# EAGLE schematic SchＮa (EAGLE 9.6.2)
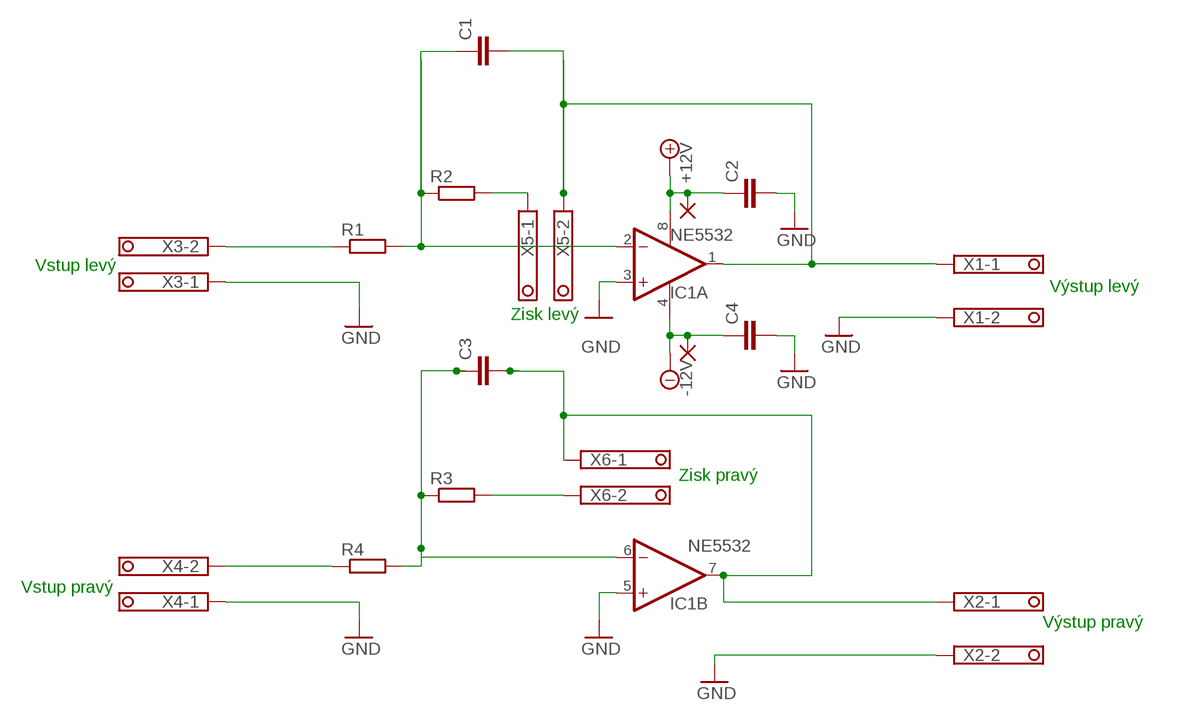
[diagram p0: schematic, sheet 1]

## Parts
+12V  1,6/0,8  [1,6/0,8]
-12V  1,6/0,8  [1,6/0,8]
C1  C-EUC1206  [C1206]
C2  C-EUC1206  [C1206]
C3  C-EUC1206  [C1206]
C4  C-EUC1206  [C1206]
IC1  NE5532  NE5532N  [DIL08]
R1  R-EU_M1206  [M1206]
R2  R-EU_M1206  [M1206]
R3  R-EU_M1206  [M1206]
R4  R-EU_M1206  [M1206]
X1  1751248  [1751248]
X2  1751248  [1751248]
X3  1751248  [1751248]
X4  1751248  [1751248]
X5  1751248  [1751248]
X6  1751248  [1751248]

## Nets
+12V: +12V.1(P) C2.1 IC1.8(P:V+)
-12V: -12V.1(P) C4.1 IC1.4(P:V-)
GND: C2.2 C4.2 IC1.3(A:+IN) IC1.5(B:+IN) X1.2 X2.2 X3.1 X4.1
N$1: C1.1 IC1.2(A:-IN) R1.2 R2.1
N$2: C3.1 IC1.6(B:-IN) R3.1 R4.2
N$3: R2.2 X5.1
N$4: R3.2 X6.2
N$5: C1.2 IC1.1(A:OUT) X1.1 X5.2
N$6: C3.2 IC1.7(B:OUT) X2.1 X6.1
N$7: R1.1 X3.2
N$8: R4.1 X4.2

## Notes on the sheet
- Vstup levý
- Výstup levý
- Zisk levý
- Zisk pravý
- Vstup pravý
- Výstup pravý

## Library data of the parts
+12V -12V = wirepad:1,6/0,8: THROUGH-HOLE PAD
C1-C4 = rcl:C-EU: CAPACITOR, European symbol; SPICEPREFIX: C
IC1 = linear:NE5532: AUDIO AMPLIFIER
R1-R4 = rcl:R-EU_: RESISTOR, European symbol; SPICEPREFIX: R
X1-X6 = con-phoenix-350:1751248: MKDS 1/ 2-3,5 Printklemme; OC_FARNELL: unknown; OC_NEWARK: unknown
